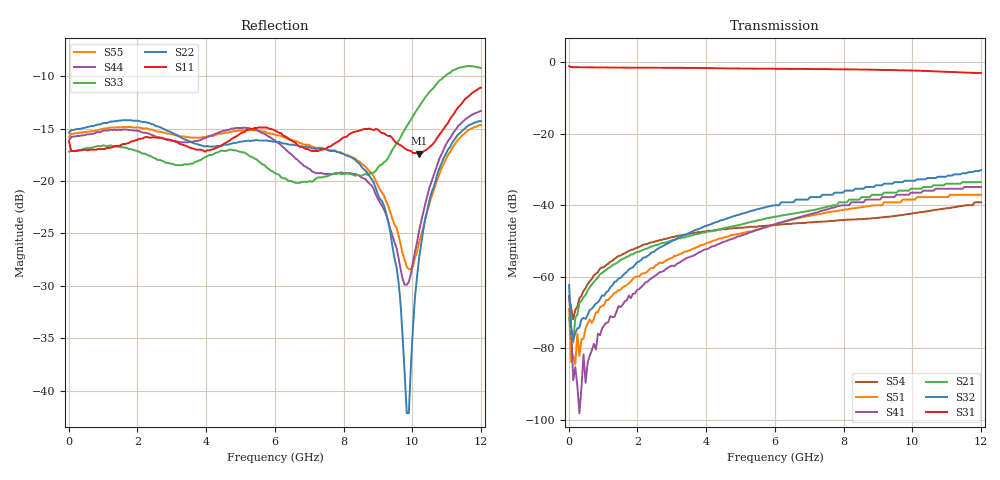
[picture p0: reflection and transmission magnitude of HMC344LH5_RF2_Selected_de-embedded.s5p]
! Hittite Microwave Corporation
! 20 Alpha Road
! Chelmsford, MA 01824
! Tel: 978-250-3343
! Fax: 978-250-3373
! Device: HMC344LH5, DC-12 GHz GaAs MMIC SP4T Non-Reflective Switch in Hermetic Leadless SMT Package
! Misc: Data was de-embedded to package pins.
!  Port 1 = RFC
!  Port 2 = RF1
!  Port 3 = RF2
!  Port 4 = RF3
!  Port 5 = RF4
!  RF2 selected, Vctl= 0/-5 V
!  Data reformated to new Touchstone file format - Tue Jan 09 13:44:54 2007
# MHz S DB R 50
! 5 Port Network Data
! freq  dbS11  angS11  dbS12  angS12  dbS13  angS13  dbS14  angS14
!  dbS15  angS15
!  dbS21  angS21  dbS22  angS22  dbS23  angS23
!  dbS24  angS24  dbS25  angS25
!  dbS31  angS31  dbS32  angS32
!  dbS33  angS33  dbS34  angS34  dbS35  angS35
!  dbS41  angS41
!  dbS42  angS42  dbS43  angS43  dbS44  angS44  dbS45  angS45
!  dbS51  angS51  dbS52  angS52  dbS53  angS53  dbS54  angS54
!  dbS55  angS55
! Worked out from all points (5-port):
!   201 points, 10 MHz to 12 GHz, reference 50 ohm
!   strongest paths, dB at 10 MHz, 3.007 GHz, 6.005 GHz, 9.002 GHz, 12 GHz:
!     S31: -1.2, -1.6, -1.9, -2.2, -3.0
!     S32: -62.3, -49.9, -40.0, -34.4, -30.2
!     S21: -71.6, -49.9, -43.2, -37.1, -33.6
!     S41: -65.4, -56.8, -45.3, -38.4, -34.9
!     S51: -68.9, -54.7, -45.3, -40.0, -37.1
!     S54: -65.3, -48.9, -45.5, -43.5, -39.2
!   lowest |S11| = -17.4 dB at 10.2 GHz (marker M1), VSWR 1.31, Z = 58.4 + j12.1 ohm
!   |S11| at or under -10 dB: start of sweep to end of sweep
